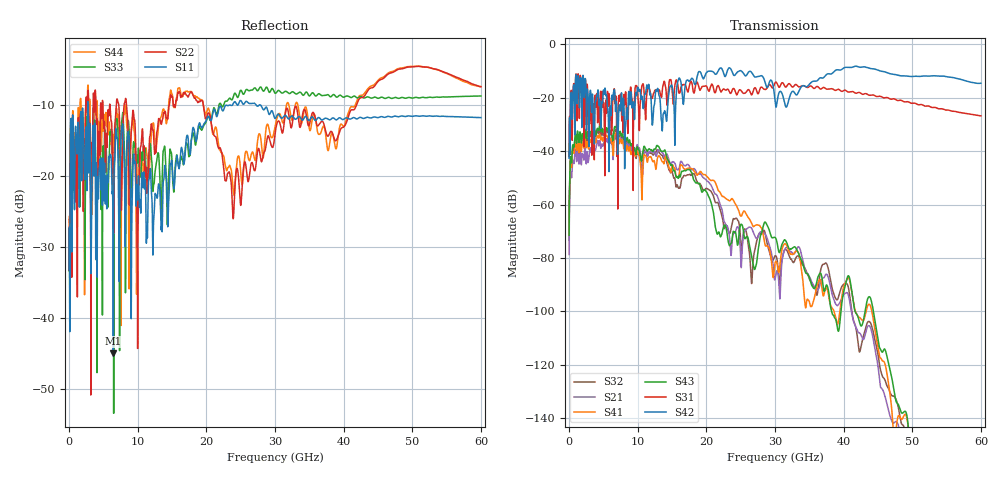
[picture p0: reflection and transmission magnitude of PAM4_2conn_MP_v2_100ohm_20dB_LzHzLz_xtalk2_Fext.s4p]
! Info: Touchstone file created by Circ.  Input file=FAB50GbE_2conn_Midplane_Examax_Topo2_v2_100ohm_20dB_LzHzLz.circ
# Hz S RI R 50
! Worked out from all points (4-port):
!   6000 points, 10 MHz to 60 GHz, reference 50 ohm
!   strongest paths, dB at 10 MHz, 15.01 GHz, 30.01 GHz, 45.01 GHz, 60 GHz:
!     S42: -42.6, -15.7, -21.2, -9.7, -14.6
!     S31: -42.1, -17.0, -14.4, -19.5, -26.8
!     S43: -71.5, -45.2, -72.3, -110.5, -155.6
!     S41: -70.8, -45.6, -82.0, -113.5, -165.4
!     S21: -78.7, -44.0, -87.9, -120.6, -161.7
!     S32: -73.4, -47.6, -79.2, -116.1, -158.6
!   lowest |S11| = -45.0 dB at 6.45 GHz (marker M1), VSWR 1.01, Z = 49.6 - j0.365 ohm
!   |S11| at or under -10 dB: start of sweep to 2.716 GHz; 2.779 GHz to 23.37 GHz (20.59 GHz wide, 157 % of centre); 27.9 GHz to end of sweep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
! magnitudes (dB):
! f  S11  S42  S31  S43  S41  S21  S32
! 10 MHz  -33.2  -42.6  -42.1  -71.5  -70.8  -78.7  -73.4
! 1.06 GHz  -14.9  -12.2  -11.9  -36.2  -38.7  -42.4  -38.0
! 6.45 GHz  -45.0  -18.4  -19.7  -35.5  -41.7  -41.5  -36.1
! 17.61 GHz  -16.9  -13.6  -14.5  -46.9  -46.5  -46.1  -48.6
! 26.91 GHz  -9.7  -11.9  -16.9  -83.5  -68.2  -70.9  -79.0
! 28.61 GHz  -10.4  -14.7  -16.9  -66.6  -75.4  -71.3  -71.2
! 60 GHz  -11.8  -14.6  -26.8  -155.6  -165.4  -161.7  -158.6
